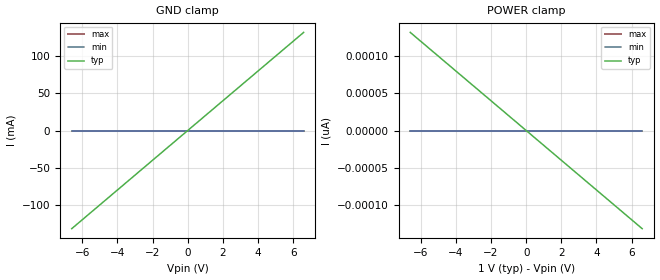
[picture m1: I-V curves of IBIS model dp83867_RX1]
[IBIS Ver]   5.1
[File Name]   dp83867_RX1.ibs
[File Rev]   1.0
[Component]   dp83867_RX1
[Manufacturer] My Company
[Package]
R_pkg  0.0   NA   NA
L_pkg  0.0   NA   NA
C_pkg  0.0   NA   NA
[Pin]   signal_name   model_name   R_pin L_pin  C_pin
2p   dp83867_RX1_2p   dp83867_RX1
2n   dp83867_RX1_2n   dp83867_RX1
[Diff_Pin] inv_pin vdiff tdelay_typ tdelay_min tdelay_max
2p   2n   NA   NA   NA   NA
| Models and submodels in the file (1): dp83867_RX1 (Input)
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[Model] dp83867_RX1
Model_type Input
C_comp 0p 0p 0p
Vinh = 0.25
Vinl = -0.25
[Temperature_Range] 25 125 0
[Voltage Range] 1.0 1.0 1.0
[Algorithmic Model]
Executable Windows_cl17.00.50727.1_64 dp83867_RX1_x64.dll dp83867_RX1.ami
Executable Windows_cl17.00.50727.1_32 dp83867_RX1.dll dp83867_RX1.ami
[End Algorithmic Model]
[GND Clamp]
-6.6V     -132mA     0A         0A
0V        0A         0A         0A
6.6V      132mA      0A         0A
[Power Clamp]
-6.6V     132pA      0A         0A
0V        0A         0A         0A
6.6V      -132pA     0A         0A
